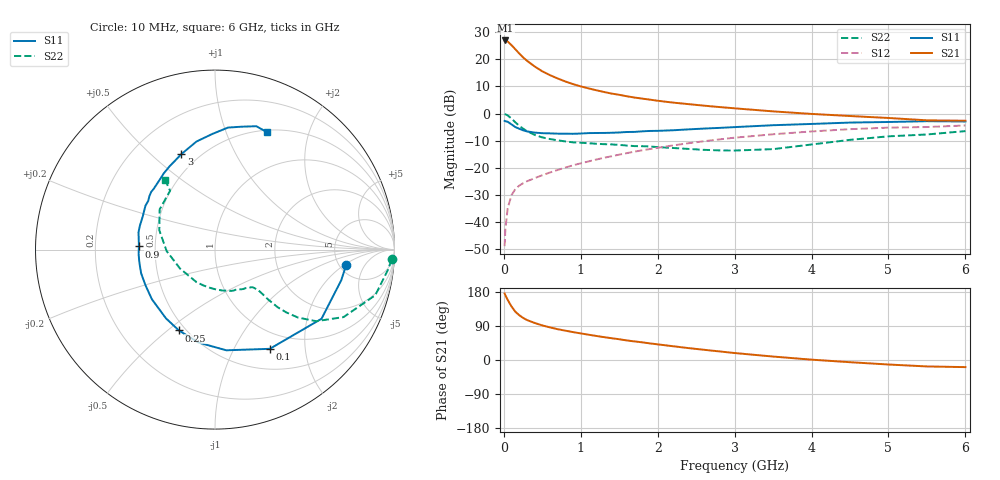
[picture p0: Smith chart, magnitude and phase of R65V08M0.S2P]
! SIEMENS Small Signal Semiconductors
! BFR193
! Si NPN RF Bipolar Junction Transistor in SOT23
! VCE = 5 V  IC = 8 mA
! Common Emitter S-Parameters:  May  1996
# GHz  S  MA  R  50
!  f  S11  S21  S12  S22
! GHz  MAG  ANG  MAG  ANG  MAG  ANG  MAG  ANG
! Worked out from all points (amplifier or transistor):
!   36 points, 10 MHz to 6 GHz, reference 50 ohm
!   highest |S21| = 27.0 dB at 20 MHz (marker M1)
!   |S21| within 3 dB of that: start of sweep to 141.5 MHz
!   unconditionally stable (mu >= 1): 789.3 MHz to 1.895 GHz; 1.922 GHz to 2.022 GHz
!   at 250 MHz: K = 0.57, MSG = 23.2 dB, |S12| = -25.7 dB
!   at 1.4 GHz: K = 1.05, MAG = 10.2 dB, |S12| = -15.7 dB
!   at 6 GHz: K = 0.95, MSG = 0.9 dB, |S12| = -4.4 dB
!   lowest NFmin = 1.25 dB at 450 MHz
!   S11 on the Smith chart (normalised r, x): 10 MHz: 5.74, -2.15; 100 MHz: 0.76, -1.40; 250 MHz: 0.46, -0.55; 900 MHz: 0.40, +0.02; 3 GHz: 0.40, +0.63; 6 GHz: 0.52, +1.41
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0.01  0.7357 -6.7  22.24 175.6  0.0036 85.8  0.9852 -3.2
0.02  0.7239 -13.6  22.32 170.8  0.0074 84.3  0.9707 -6.6
0.05  0.7076 -33.0  21.3 158.5  0.0181 74.5  0.9283 -15.9
0.1  0.6315 -61.1  18.27 141.2  0.0314 64.2  0.8089 -27.7
0.15  0.5645 -83.6  15.34 127.3  0.0408 57.9  0.6904 -35.3
0.2  0.526 -100.1  12.87 118.3  0.047 54.8  0.5978 -39.3
0.25  0.4931 -114.1  10.89 111.2  0.052 53.0  0.5283 -41.4
0.3  0.4705 -125.5  9.453 105.5  0.0565 53.7  0.4757 -42.6
0.4  0.4474 -141.8  7.415 97.8  0.0646 54.5  0.4052 -43.2
0.5  0.4355 -152.8  6.015 91.3  0.0732 56.0  0.3643 -43.1
0.6  0.4322 -162.4  5.114 86.0  0.0822 57.3  0.34 -43.1
0.7  0.4274 -170.5  4.444 81.3  0.0916 58.9  0.3218 -43.6
0.9  0.4245 177.6  3.495 73.6  0.1116 60.4  0.2956 -45.1
1.1  0.4371 167.2  2.92 66.8  0.1313 61.2  0.2847 -48.3
1.3  0.4403 158.8  2.508 60.4  0.1533 61.1  0.2734 -51.8
1.6  0.4583 147.6  2.087 51.6  0.1868 60.0  0.2578 -59.3
2.2  0.4932 129.5  1.596 36.3  0.2596 55.4  0.2325 -79.0
3  0.564 109.4  1.252 18.4  0.3599 45.5  0.2084 -119.9
3.5  0.6111 99.7  1.1 9.1  0.4161 37.9  0.2215 -151.4
4.5  0.6838 83.9  0.903 -5.8  0.5166 22.6  0.3283 160.9
5.5  0.7249 71.5  0.752 -17.0  0.5659 6.6  0.4125 127.3
6  0.7155 66.0  0.739 -18.8  0.6049 2.0  0.4758 125.7
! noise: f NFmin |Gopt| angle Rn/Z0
0.45  1.25  0.23  133  0.12
0.9  1.3  0.35  156  0.11
1.8  2  0.55  -155  0.13
